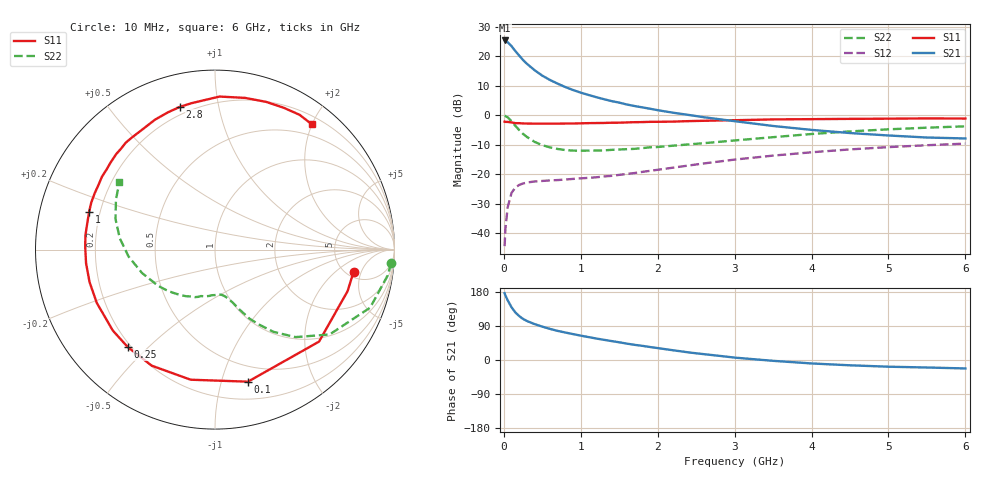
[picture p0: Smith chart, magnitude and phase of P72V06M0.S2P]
! SIEMENS Small Signal Semiconductors
! BFP196
! Si NPN RF Bipolar Junction Transistor in SOT143
! VCE = 2 V  IC = 6 mA
! Common Emitter S-Parameters:  May  1996
# GHz  S  MA  R  50
!  f  S11  S21  S12  S22
! GHz  MAG  ANG  MAG  ANG  MAG  ANG  MAG  ANG
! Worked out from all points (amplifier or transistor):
!   36 points, 10 MHz to 6 GHz, reference 50 ohm
!   highest |S21| = 25.3 dB at 10 MHz (marker M1)
!   |S21| within 3 dB of that: start of sweep to 132.1 MHz
!   unconditionally stable (mu >= 1): 1.055 GHz to 3.262 GHz
!   at 250 MHz: K = 0.29, MSG = 20.9 dB, |S12| = -23.1 dB
!   at 1.4 GHz: K = 1.16, MAG = 10.2 dB, |S12| = -20.5 dB
!   at 6 GHz: K = 1.00, MSG = 0.9 dB, |S12| = -9.6 dB
!   S11 on the Smith chart (normalised r, x): 10 MHz: 5.82, -3.66; 100 MHz: 0.35, -1.22; 250 MHz: 0.19, -0.43; 1 GHz: 0.16, +0.14; 2.8 GHz: 0.16, +0.77; 6 GHz: 0.32, +1.99
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0.01  0.782 -9.0  18.5 176.3  0.0061 86.9  0.9843 -4.4
0.02  0.7742 -17.4  18.17 170.4  0.0119 81.9  0.9728 -8.5
0.05  0.7738 -41.5  17.24 157.5  0.0279 69.6  0.923 -20.5
0.1  0.7584 -76.0  14.82 139.2  0.0486 54.5  0.7948 -36.5
0.15  0.7375 -100.6  12.23 125.4  0.06 43.4  0.6623 -47.4
0.2  0.7365 -118.6  10.26 115.9  0.0664 36.9  0.5621 -54.6
0.25  0.7288 -131.9  8.628 108.4  0.0702 32.0  0.485 -59.5
0.3  0.7263 -141.6  7.45 102.9  0.0729 29.2  0.4305 -63.4
0.4  0.7225 -155.8  5.799 94.7  0.0759 25.9  0.3552 -68.2
0.5  0.722 -165.5  4.695 88.0  0.0775 24.3  0.3128 -71.4
0.6  0.7224 -174.0  3.965 82.1  0.0791 24.4  0.2862 -74.4
0.7  0.7229 179.3  3.432 76.8  0.0802 24.6  0.2694 -77.3
0.8  0.7265 173.8  3.01 72.5  0.082 25.1  0.2583 -80.2
1  0.732 163.5  2.42 64.3  0.0857 27.4  0.2522 -85.2
1.1  0.7376 159.2  2.212 60.5  0.0874 28.6  0.2529 -88.2
1.6  0.758 139.9  1.523 43.2  0.1018 35.5  0.2675 -103.9
2.2  0.7826 120.8  1.107 25.7  0.1301 39.4  0.3062 -122.0
2.8  0.8189 103.8  0.86 11.0  0.1653 38.1  0.356 -141.3
3.5  0.8531 88.3  0.66 -2.2  0.2079 32.2  0.4269 -162.2
4.5  0.871 70.9  0.501 -14.0  0.265 21.1  0.5344 173.2
5.5  0.8867 57.9  0.421 -19.8  0.3119 9.0  0.6178 153.3
6  0.8821 52.4  0.406 -22.3  0.3323 2.5  0.6517 144.8
